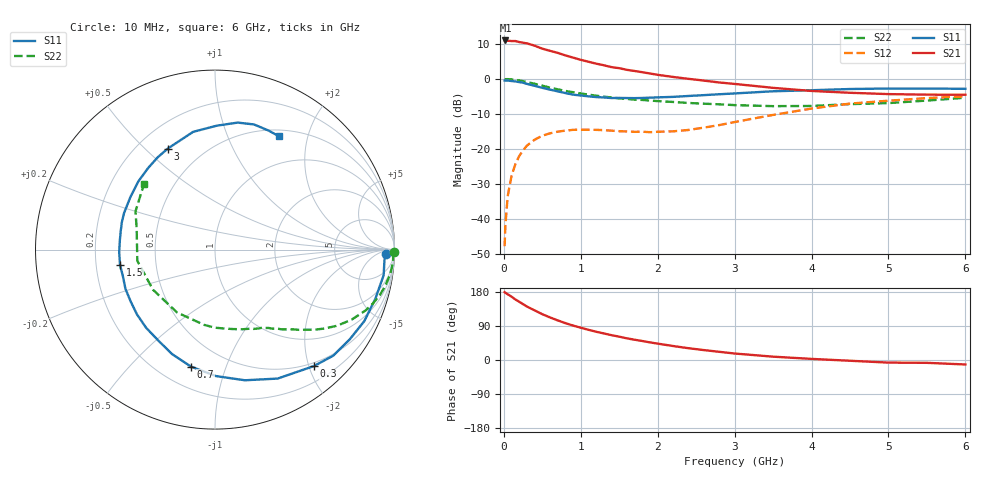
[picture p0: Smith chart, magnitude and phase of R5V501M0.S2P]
! SIEMENS Small Signal Semiconductors
! BFR183
! Si NPN RF Bipolar Junction Transistor in SOT23
! VCE = 0.5 V  IC = 1 mA
! Common Emitter S-Parameters:  May  1996
# GHz  S  MA  R  50
!  f  S11  S21  S12  S22
! GHz  MAG  ANG  MAG  ANG  MAG  ANG  MAG  ANG
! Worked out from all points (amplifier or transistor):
!   36 points, 10 MHz to 6 GHz, reference 50 ohm
!   highest |S21| = 11.0 dB at 20 MHz (marker M1)
!   |S21| within 3 dB of that: start of sweep to 606.5 MHz
!   unconditionally stable (mu >= 1): 1.574 GHz to 4.064 GHz; 5.066 GHz to end of sweep
!   at 250 MHz: K = 0.17, MSG = 15.4 dB, |S12| = -20.4 dB
!   at 1.4 GHz: K = 0.91, MSG = 9.1 dB, |S12| = -14.8 dB
!   at 6 GHz: K = 1.02, MAG = -0.6 dB, |S12| = -4.9 dB
!   S11 on the Smith chart (normalised r, x): 10 MHz: 30, -17; 300 MHz: 0.44, -2.08; 700 MHz: 0.33, -0.76; 1.5 GHz: 0.30, -0.07; 3 GHz: 0.32, +0.59; 6 GHz: 0.58, +1.56
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0.01  0.9506 -1.6  3.508 179.1  0.0041 88.6  0.9969 -0.8
0.02  0.9459 -3.5  3.547 177.3  0.0081 86.4  0.9931 -1.5
0.05  0.9504 -8.6  3.512 173.5  0.0211 84.1  0.9943 -4.0
0.1  0.9345 -17.1  3.479 167.1  0.0414 79.4  0.9857 -7.9
0.15  0.9224 -25.6  3.477 159.7  0.0608 74.2  0.9712 -11.7
0.3  0.8511 -49.7  3.224 141.1  0.1115 60.5  0.9059 -21.9
0.4  0.7988 -64.1  2.986 131.0  0.1357 52.6  0.8549 -27.2
0.5  0.7469 -77.1  2.706 120.9  0.1547 45.7  0.8022 -31.9
0.7  0.6654 -101.6  2.358 104.5  0.1768 35.3  0.7121 -38.8
0.8  0.6295 -112.3  2.171 97.3  0.183 31.4  0.6749 -41.4
0.9  0.5971 -121.9  2.017 90.9  0.1878 28.2  0.6472 -43.7
1.1  0.5652 -140.2  1.761 79.7  0.1888 23.4  0.5976 -48.1
1.3  0.5446 -156.4  1.569 70.1  0.1858 20.6  0.5586 -51.9
1.5  0.536 -171.0  1.426 61.6  0.1796 20.3  0.5282 -55.7
1.9  0.541 163.6  1.196 46.4  0.1739 23.8  0.4921 -63.9
2.2  0.5551 148.0  1.069 36.9  0.1788 29.5  0.4695 -71.0
3  0.6215 115.0  0.85 17.1  0.2427 40.5  0.4235 -98.3
3.5  0.6673 100.5  0.747 8.8  0.3069 39.2  0.4092 -121.1
4.5  0.7188 79.9  0.635 -2.0  0.4448 26.6  0.4373 -171.8
5  0.7303 72.7  0.608 -6.9  0.4895 17.4  0.4525 164.7
5.5  0.7273 65.9  0.597 -7.5  0.5334 11.9  0.4916 154.3
6  0.7252 60.5  0.596 -11.8  0.566 2.9  0.5397 137.0
